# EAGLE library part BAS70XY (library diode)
Silicon Schottky Diodes General-purpose diode for high-speed switching Source: BAS70_1PS7XSB70_SER_8.pdf
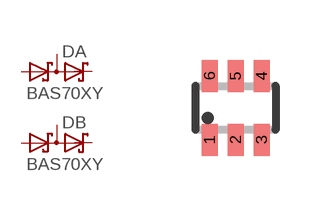
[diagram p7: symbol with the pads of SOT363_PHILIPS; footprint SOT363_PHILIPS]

Designator prefix D; gates A=SDD_AKAK B=SDD_AKAK

## BAS70XY  [SOT363_PHILIPS]
1  A:A1  pas
2  A:C2  pas
3  B:C1A2  pas
4  B:A1  pas
5  B:C2  pas
6  A:C1A2  pas

## Footprint SOT363_PHILIPS (pad centres in mm)
Small Outline Transistor; 6 leads Philips Semiconductors, SOT363.pdf
smd 0.4 x 0.8: 1 -0.65,-0.8; 2 0,-0.8; 3 0.65,-0.8; 4 0.65,0.8; 5 0,0.8; 6 -0.65,0.8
